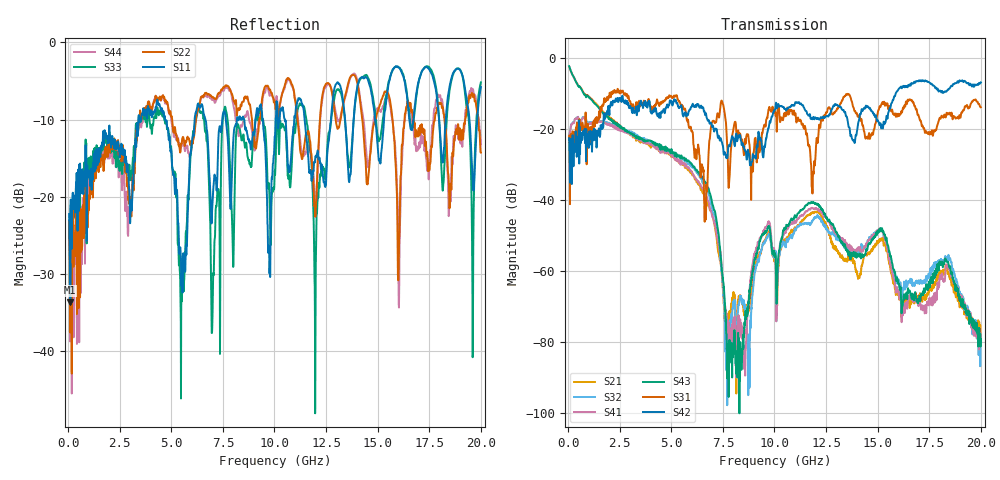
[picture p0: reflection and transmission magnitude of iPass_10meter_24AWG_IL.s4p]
! FILE: D:\iPass\iPassCables1205\10meter\iPass_10meter_24AWG_IL.s4p
# MHz S MA R 50.00
! FREQ  S11  S12  S13  S14
!  S21  S22  S23  S24
!  S31  S32  S33  S34
!  S41  S42  S43  S44
!  MAG  ANG  MAG  ANG  MAG  ANG  MAG  ANG
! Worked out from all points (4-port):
!   1996 points, 50 MHz to 20 GHz, reference 50 ohm
!   strongest paths, dB at 50 MHz, 5.04 GHz, 10.03 GHz, 15.02 GHz, 20 GHz:
!     S42: -22.5, -13.0, -14.3, -17.8, -6.8
!     S31: -21.8, -11.1, -15.1, -14.8, -13.8
!     S43: -2.2, -26.7, -55.9, -49.0, -79.7
!     S41: -23.6, -27.6, -55.3, -48.7, -79.1
!     S32: -23.6, -26.7, -54.2, -48.7, -80.6
!     S21: -2.2, -27.3, -56.9, -51.7, -79.6
!   lowest |S11| = -33.7 dB at 110 MHz (marker M1), VSWR 1.04, Z = 51.7 - j1.28 ohm
!   |S11| at or under -10 dB: start of sweep to 3.408 GHz; 4.701 GHz to 6.13 GHz (1.429 GHz wide, 26.4 % of centre); 11.46 GHz to 12.74 GHz (1.277 GHz wide, 10.6 % of centre)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
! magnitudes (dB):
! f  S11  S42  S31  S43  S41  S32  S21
! 50 MHz  -22.2  -22.5  -21.8  -2.2  -23.6  -23.6  -2.2
! 110 MHz  -33.7  -25.6  -29.4  -3.2  -20.2  -20.0  -3.2
! 5.53 GHz  -32.3  -14.9  -13.3  -28.2  -29.8  -28.4  -29.9
! 6.18 GHz  -9.1  -13.4  -27.0  -31.2  -33.9  -31.4  -33.8
! 7.78 GHz  -14.9  -24.5  -36.5  -95.4  -79.1  -80.1  -75.8
! 11.83 GHz  -17.6  -17.1  -36.5  -40.5  -42.1  -45.9  -43.3
! 20 GHz  -5.8  -6.8  -13.8  -79.7  -79.1  -80.6  -79.6
